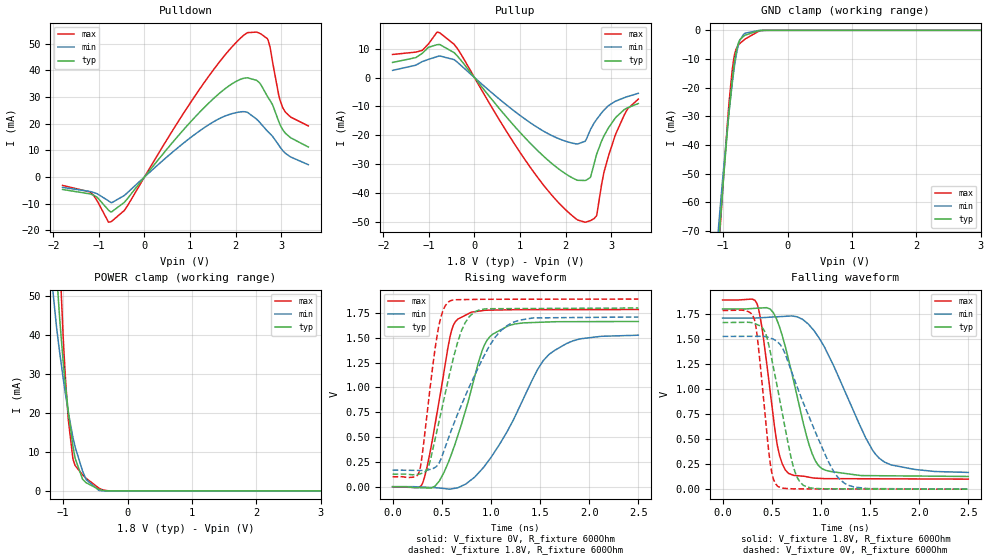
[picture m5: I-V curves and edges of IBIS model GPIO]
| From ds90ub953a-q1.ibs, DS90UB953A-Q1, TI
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|   GPIO Model
[Model]   GPIO
Model_type   I/O
Polarity   Non-Inverting
Enable   Active-Low
Vinl = 0.54
Vinh = 1.26
Vmeas = 0.9
Vref = 0
Cref = 0.1pF
Rref = 1000000
|   typ   min   max
C_comp   0.5024pF   0.4pF   0.5979pF
|C_comp_pull_up   0.3943pF   0.3332pF   0.4592pF
|C_comp_pull_down   0.3994pF   0.3369pF   0.4616pF
[Model spec]
|subparameter
Vinl   0.63   0.5985   0.6615
Vinh   1.17   1.1115   1.2285
[Voltage Range]   1.8   1.71   1.89
|Junction Temperature
[Temperature Range]   27   105   -40
[Pullup Reference]   1.8   1.71   1.89
[Pulldown Reference]   0   0   0
[Power Clamp Reference]   1.8   1.71   1.89
[GND Clamp Reference]   0   0   0
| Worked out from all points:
|   slope of the pulldown table from 0 to 0.27 V, typ, clamps not added: 46.6 ohm
|   slope of the pullup table from 0 to 0.27 V, typ, clamps not added: 50.1 ohm
|   GND clamp passes 1 mA (typ) near -0.57 V on its own axis
|   POWER clamp passes 1 mA (typ) near -0.51 V on its own axis
|   falling waveform, V_fixture 1.8V, R_fixture 600Ohm: 20-80 % time 248ps typ, 431ps min, 141ps max; typ from 1.8 V to 0.127 V
|   rising waveform, V_fixture 0V, R_fixture 600Ohm: 20-80 % time 298ps typ, 493ps min, 185ps max; typ from 0 V to 1.66 V
|   rising waveform, V_fixture 1.8V, R_fixture 600Ohm: 20-80 % time 236ps typ, 412ps min, 136ps max; typ from 0.127 V to 1.8 V
|   falling waveform, V_fixture 0V, R_fixture 600Ohm: 20-80 % time 199ps typ, 377ps min, 108ps max; typ from 1.66 V to 0 V
[Pulldown]
|   Voltage   I(typ)   I(min)   I(max)
-1.8V     -4.687mA   -3.898mA   -3.166mA
-1.19V    -6.376mA   -5.465mA   -5.641mA
-790.2mV  -12.46mA   -8.964mA   -16.97mA
-720mV    -13.06mA   -9.66mA    -16.63mA
-369mV    -8.003mA   -5.805mA   -10.66mA
1.316V    26.12mA    18.54mA    35.53mA
2.266V    37.21mA    24.23mA    54.18mA
2.515V    35.58mA    20.84mA    54.06mA
2.704V    30.21mA    17.17mA    51.78mA
2.947V    20.97mA    12.06mA    30.99mA
3.038V    17.71mA    9.891mA    25.99mA
3.6V      11.24mA    4.616mA    19.16mA
[GND Clamp]
|   Voltage   I(typ)   I(min)   I(max)
-1.8V     -338.1mA   -296.3mA   -392.2mA
-1.071V   -75.3mA    -68.41mA   -77.78mA
-1.055V   -70.12mA   -64.07mA   -71.98mA
-1.044V   -66.71mA   -61.21mA   -68.17mA
-995.4mV  -51.93mA   -48.79mA   -51.63mA
-903.6mV  -27.3mA    -27.48mA   -24.02mA
-860.4mV  -17.69mA   -18.77mA   -14.07mA
-833.4mV  -12.6mA    -13.99mA   -9.673mA
-763.2mV  -4.392mA   -5.046mA   -5.124mA
-655.2mV  -1.664mA   -988.9uA   -2.984mA
-352.8mV  -9.596uA   -7.087uA   -20.74uA
3.6V      0A         0A         0A
[Pullup]
|   Voltage   I(typ)   I(min)   I(max)
-1.8V     5.231mA    2.488mA    7.992mA
-1.147V   8.384mA    5.541mA    9.424mA
-822.6mV  11.37mA    7.259mA    15.72mA
-444.6mV  8.593mA    6.194mA    11.46mA
1.316V    -24.15mA   -16.56mA   -32.99mA
2.428V    -35.59mA   -22.06mA   -50.01mA
2.552V    -34.27mA   -17.85mA   -49.43mA
2.682V    -26.62mA   -14.5mA    -47.71mA
2.844V    -20.2mA    -11.25mA   -32.8mA
3.082V    -14.25mA   -8.312mA   -20.45mA
3.368V    -10.41mA   -6.547mA   -10.73mA
3.6V      -8.98mA    -5.446mA   -7.452mA
[POWER Clamp]
|   Voltage   I(typ)   I(min)   I(max)
-1.8V     370.4mA    281.4mA    456.9mA
-1.19V    86.55mA    56.36mA    123.6mA
-1.076V   49.76mA    38.51mA    69.59mA
-1.055V   44.49mA    35.71mA    60.41mA
-1.001V   33.4mA     29.1mA     40.07mA
-963mV    26.92mA    24.78mA    28.56mA
-919.8mV  20.37mA    20.2mA     18.28mA
-849.6mV  11.68mA    13.89mA    8.446mA
-811.8mV  8.276mA    11.19mA    6.474mA
-698.4mV  3.015mA    5.099mA    4.139mA
-444.6mV  388.9uA    137.1uA    708.7uA
3.6V      0A         0A         0A
[Ramp]
R_load = 600
|   typ   min   max
dV/dt_r   0.998369/2.96125e-10   0.914752/4.90405e-10   1.07046/1.84492e-10
dV/dt_f   1.00371/2.47536e-10   0.925122/4.28126e-10   1.07354/1.4097e-10
[Falling Waveform]
V_fixture = 1.8V
V_fixture_min = 1.71V
V_fixture_max = 1.89V
R_fixture = 600Ohm
C_fixture = 0F
|   Time   V(typ)   V(min)   V(max)
0s        1.8V       1.709V     1.89V
350.8ps   1.807V     1.71V      1.852V
413ps     1.811V     1.714V     1.528V
558.5ps   1.675V     1.722V     430.5mV
669.2ps   1.302V     1.728V     159.1mV
880.4ps   442.7mV    1.64V      119.6mV
1.01ns    205.9mV    1.463V     106.6mV
1.456ns   135.6mV    511.3mV    104.1mV
1.596ns   134.5mV    307.7mV    103.6mV
2.5ns     127mV      167.5mV    100.6mV
[Rising Waveform]
V_fixture = 0V
V_fixture_min = 0V
V_fixture_max = 0V
R_fixture = 600Ohm
C_fixture = 0F
|   Time   V(typ)   V(min)   V(max)
0s        138.1uV    1.185mV    71.65uV
306.9ps   -10.51mV   -3.618mV   39.79mV
431.2ps   5.583mV    -9.428mV   621.6mV
583.5ps   286.6mV    -24.29mV   1.506V
664.3ps   517.3mV    -9.985mV   1.688V
911.4ps   1.371V     179.3mV    1.773V
1.023ns   1.539V     328.8mV    1.779V
1.594ns   1.659V     1.334V     1.784V
1.908ns   1.662V     1.489V     1.784V
2.5ns     1.664V     1.526V     1.784V
[Rising Waveform]
V_fixture = 1.8V
V_fixture_min = 1.71V
V_fixture_max = 1.89V
R_fixture = 600Ohm
C_fixture = 0F
|   Time   V(typ)   V(min)   V(max)
0s        126.8mV    167.3mV    100.5mV
272.6ps   127.5mV    164.6mV    153mV
359.3ps   187.2mV    168.5mV    804.4mV
455.9ps   583.5mV    214.5mV    1.54V
571.5ps   1.098V     498.4mV    1.863V
700.9ps   1.571V     823.4mV    1.884V
781.9ps   1.714V     1.01V      1.885V
981.2ps   1.793V     1.411V     1.888V
1.171ns   1.793V     1.626V     1.888V
2.5ns     1.8V       1.709V     1.89V
[Falling Waveform]
|Gnd
V_fixture = 0V
V_fixture_min = 0V
V_fixture_max = 0V
R_fixture = 600Ohm
C_fixture = 0F
|   Time   V(typ)   V(min)   V(max)
0s        1.664V     1.526V     1.784V
321.9ps   1.656V     1.527V     1.701V
428.2ps   1.577V     1.525V     789.1mV
484.9ps   1.374V     1.51V      258.5mV
562.5ps   991.1mV    1.468V     27.36mV
708.9ps   266.3mV    1.155V     3.75mV
789.9ps   68.13mV    941.6mV    3.148mV
1.11ns    3.336mV    210.2mV    2.598mV
1.242ns   3.046mV    58.2mV     2.371mV
2.5ns     280.5uV    1.336mV    211.3uV
